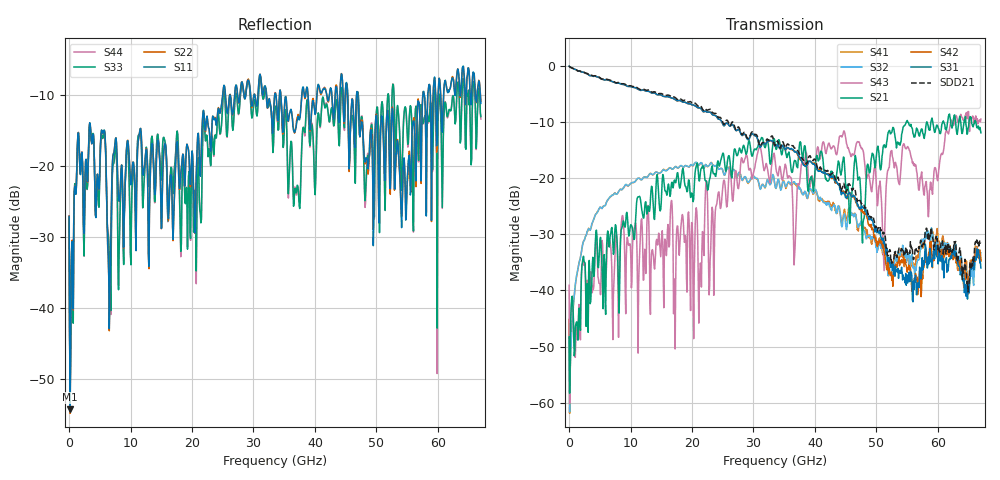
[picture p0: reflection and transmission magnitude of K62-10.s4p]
!Agilent Technologies,N5247A,US50470101,A.10.25.02
!Agilent N5247A: A.10.25.02
!Date: Tuesday, May 12, 2015 13:40:09
!Correction: Sdd11(Full 4 Port(1,2,3,4))
!Sdc11(Full 4 Port(1,2,3,4))
!Sdd12(Full 4 Port(1,2,3,4))
!Sdc12(Full 4 Port(1,2,3,4))
!Scd11(Full 4 Port(1,2,3,4))
!Scc11(Full 4 Port(1,2,3,4))
!Scd12(Full 4 Port(1,2,3,4))
!Scc12(Full 4 Port(1,2,3,4))
!Sdd21(Full 4 Port(1,2,3,4))
!Sdc21(Full 4 Port(1,2,3,4))
!Sdd22(Full 4 Port(1,2,3,4))
!Sdc22(Full 4 Port(1,2,3,4))
!Scd21(Full 4 Port(1,2,3,4))
!Scc21(Full 4 Port(1,2,3,4))
!Scd22(Full 4 Port(1,2,3,4))
!Scc22(Full 4 Port(1,2,3,4))
!Balanced Topology: BBAL
!S4P File: Measurements: <Sdd11,Sdc11,Sdd12,Sdc12>,
!<Scd11,Scc11,Scd12,Scc12>,
!<Sdd21,Sdc21,Sdd22,Sdc22>,
!<Scd21,Scc21,Scd22,Scc22>:
# Hz S  dB  R 50
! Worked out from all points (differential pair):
!   801 points, 10 MHz to 67 GHz, reference 50 ohm
!   strongest paths, dB at 10 MHz, 16.76 GHz, 33.51 GHz, 50.25 GHz, 67 GHz:
!     S31: 0.0, -5.7, -14.3, -29.7, -36.0
!     S42: 0.0, -5.7, -14.2, -31.3, -34.7
!     S21: -48.3, -20.7, -13.6, -14.3, -11.9
!     S43: -39.1, -24.7, -16.7, -24.1, -9.4
!     S32: -48.9, -18.4, -21.4, -32.6, -33.3
!     S41: -45.2, -18.4, -21.2, -32.1, -34.7
!   taken as a pair (ports 1,2 in; 3,4 out), SDD21 dB: 0.0, -5.4, -14.1, -28.8, -31.6
!   lowest |S11| = -54.2 dB at 177.5 MHz (marker M1), VSWR 1.00, Z = 49.8 - j0.111 ohm
!   |S11| at or under -10 dB: start of sweep to 24.99 GHz; 34.45 GHz to 37.86 GHz (3.41 GHz wide, 9.43 % of centre); 46.99 GHz to 57.57 GHz (10.58 GHz wide, 20.2 % of centre)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
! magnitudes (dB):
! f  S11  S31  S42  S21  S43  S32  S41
! 10 MHz  -27.1  0.0  0.0  -48.3  -39.1  -48.9  -45.2
! 177.5 MHz  -54.2  -0.2  -0.2  -51.3  -51.0  -53.9  -54.8
! 3.611 GHz  -16.3  -1.7  -1.7  -39.8  -37.2  -28.7  -28.7
! 6.542 GHz  -42.9  -2.5  -2.6  -32.3  -31.1  -23.5  -23.5
! 7.463 GHz  -16.9  -2.9  -3.0  -29.1  -33.7  -22.6  -22.6
! 16.34 GHz  -23.9  -5.5  -5.5  -22.6  -31.9  -18.2  -18.1
! 67 GHz  -11.2  -36.0  -34.7  -11.9  -9.4  -33.3  -34.7
